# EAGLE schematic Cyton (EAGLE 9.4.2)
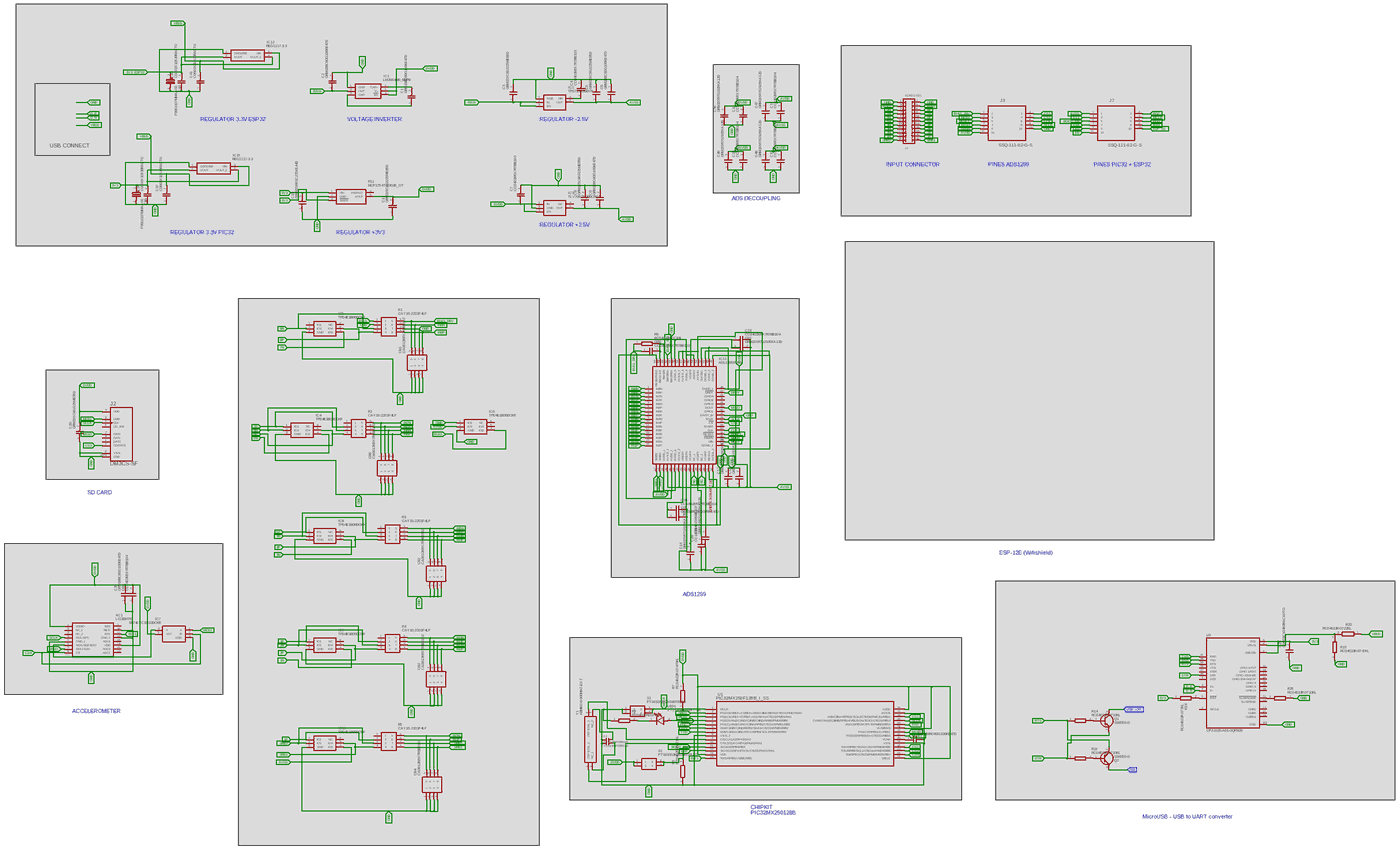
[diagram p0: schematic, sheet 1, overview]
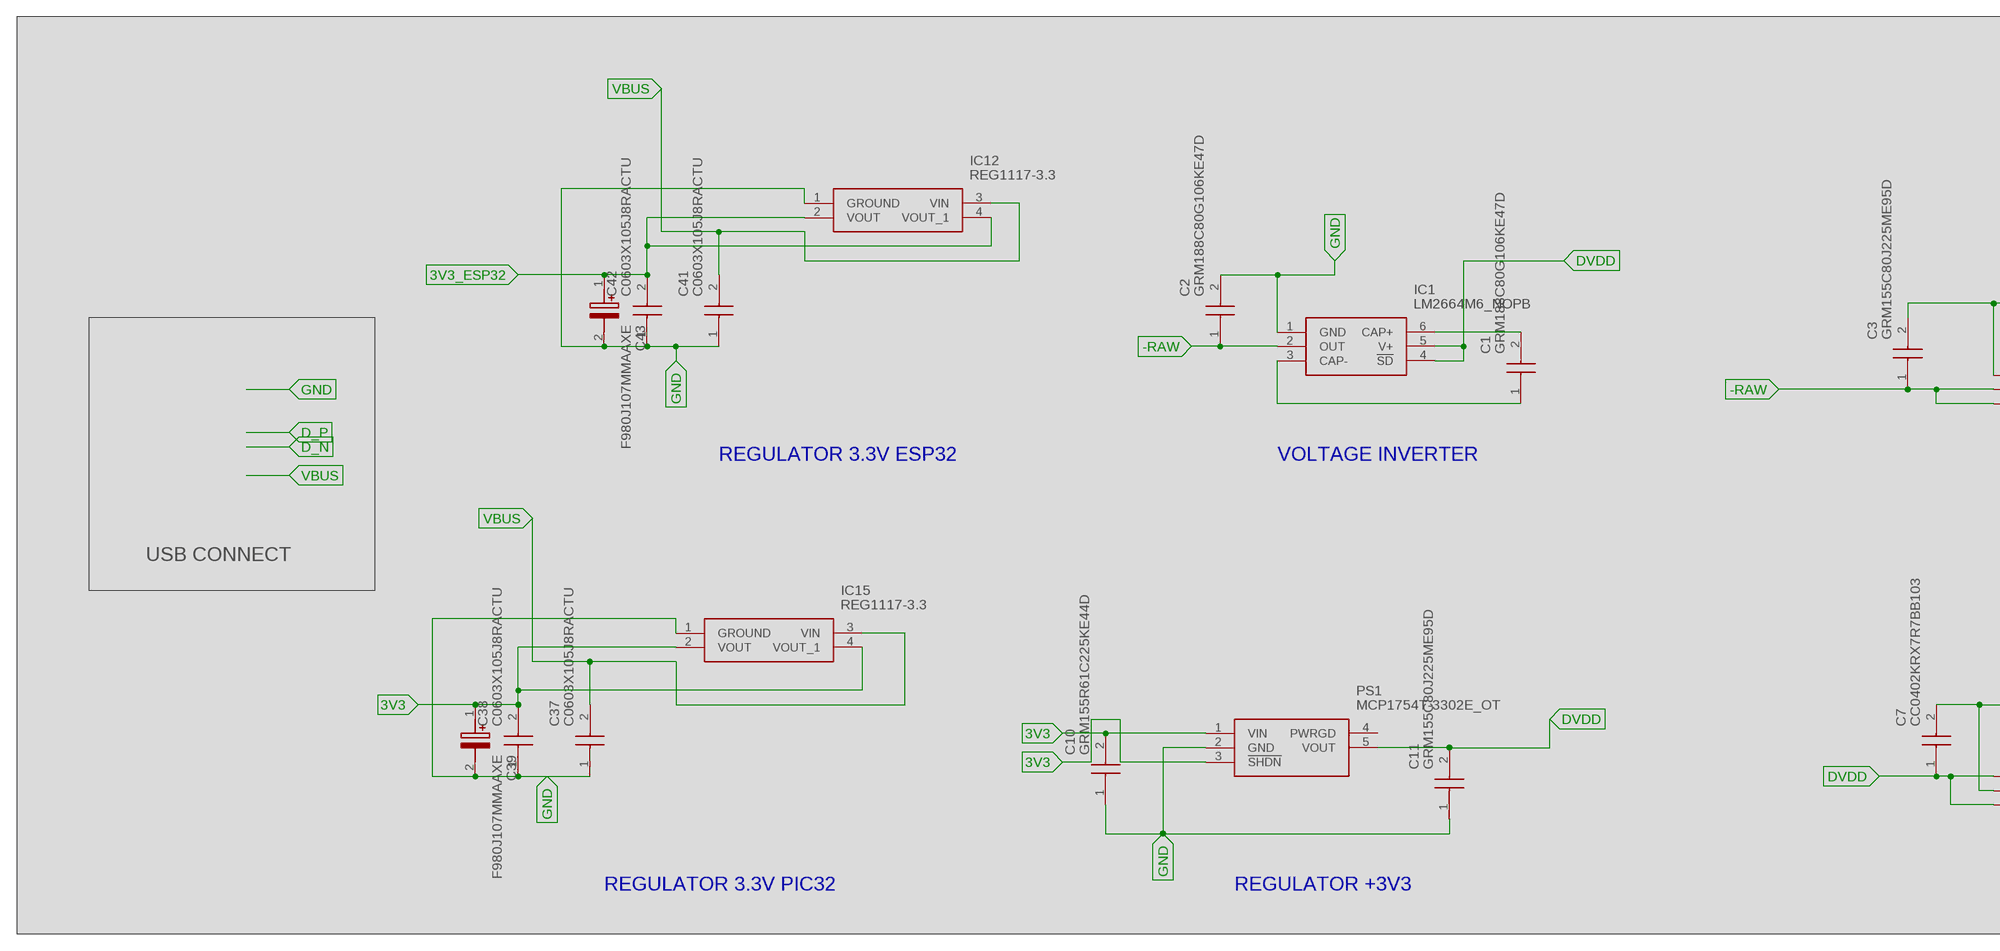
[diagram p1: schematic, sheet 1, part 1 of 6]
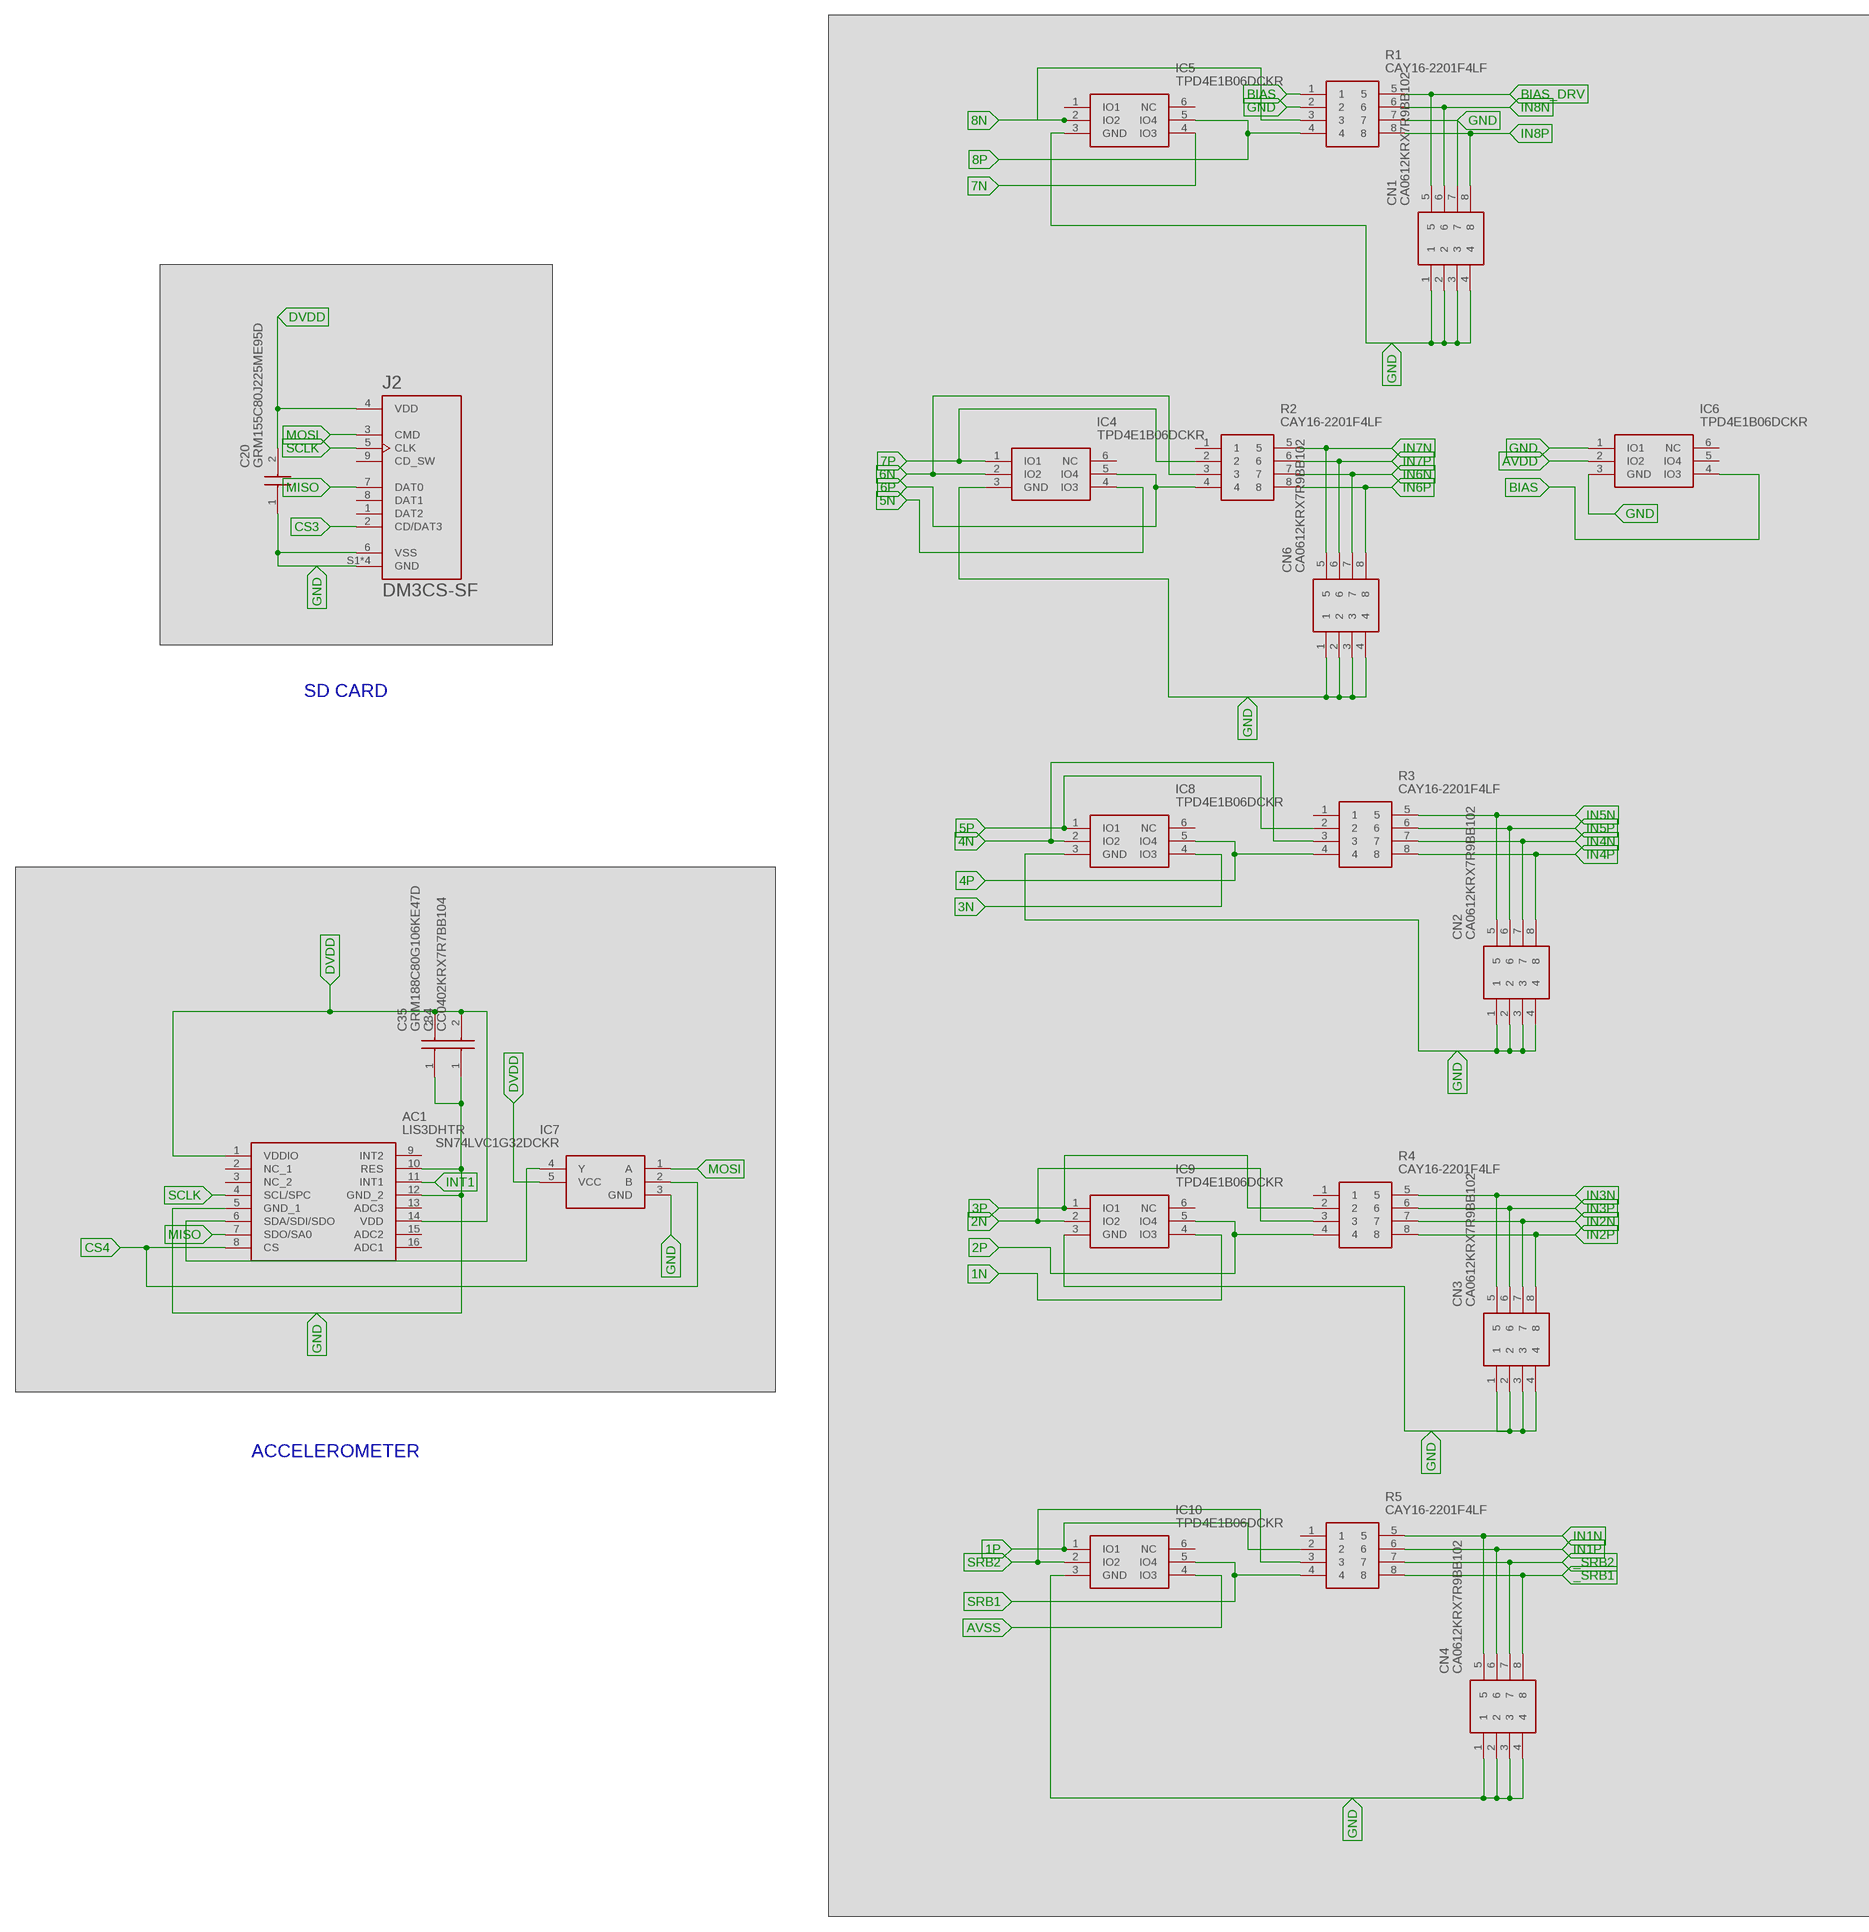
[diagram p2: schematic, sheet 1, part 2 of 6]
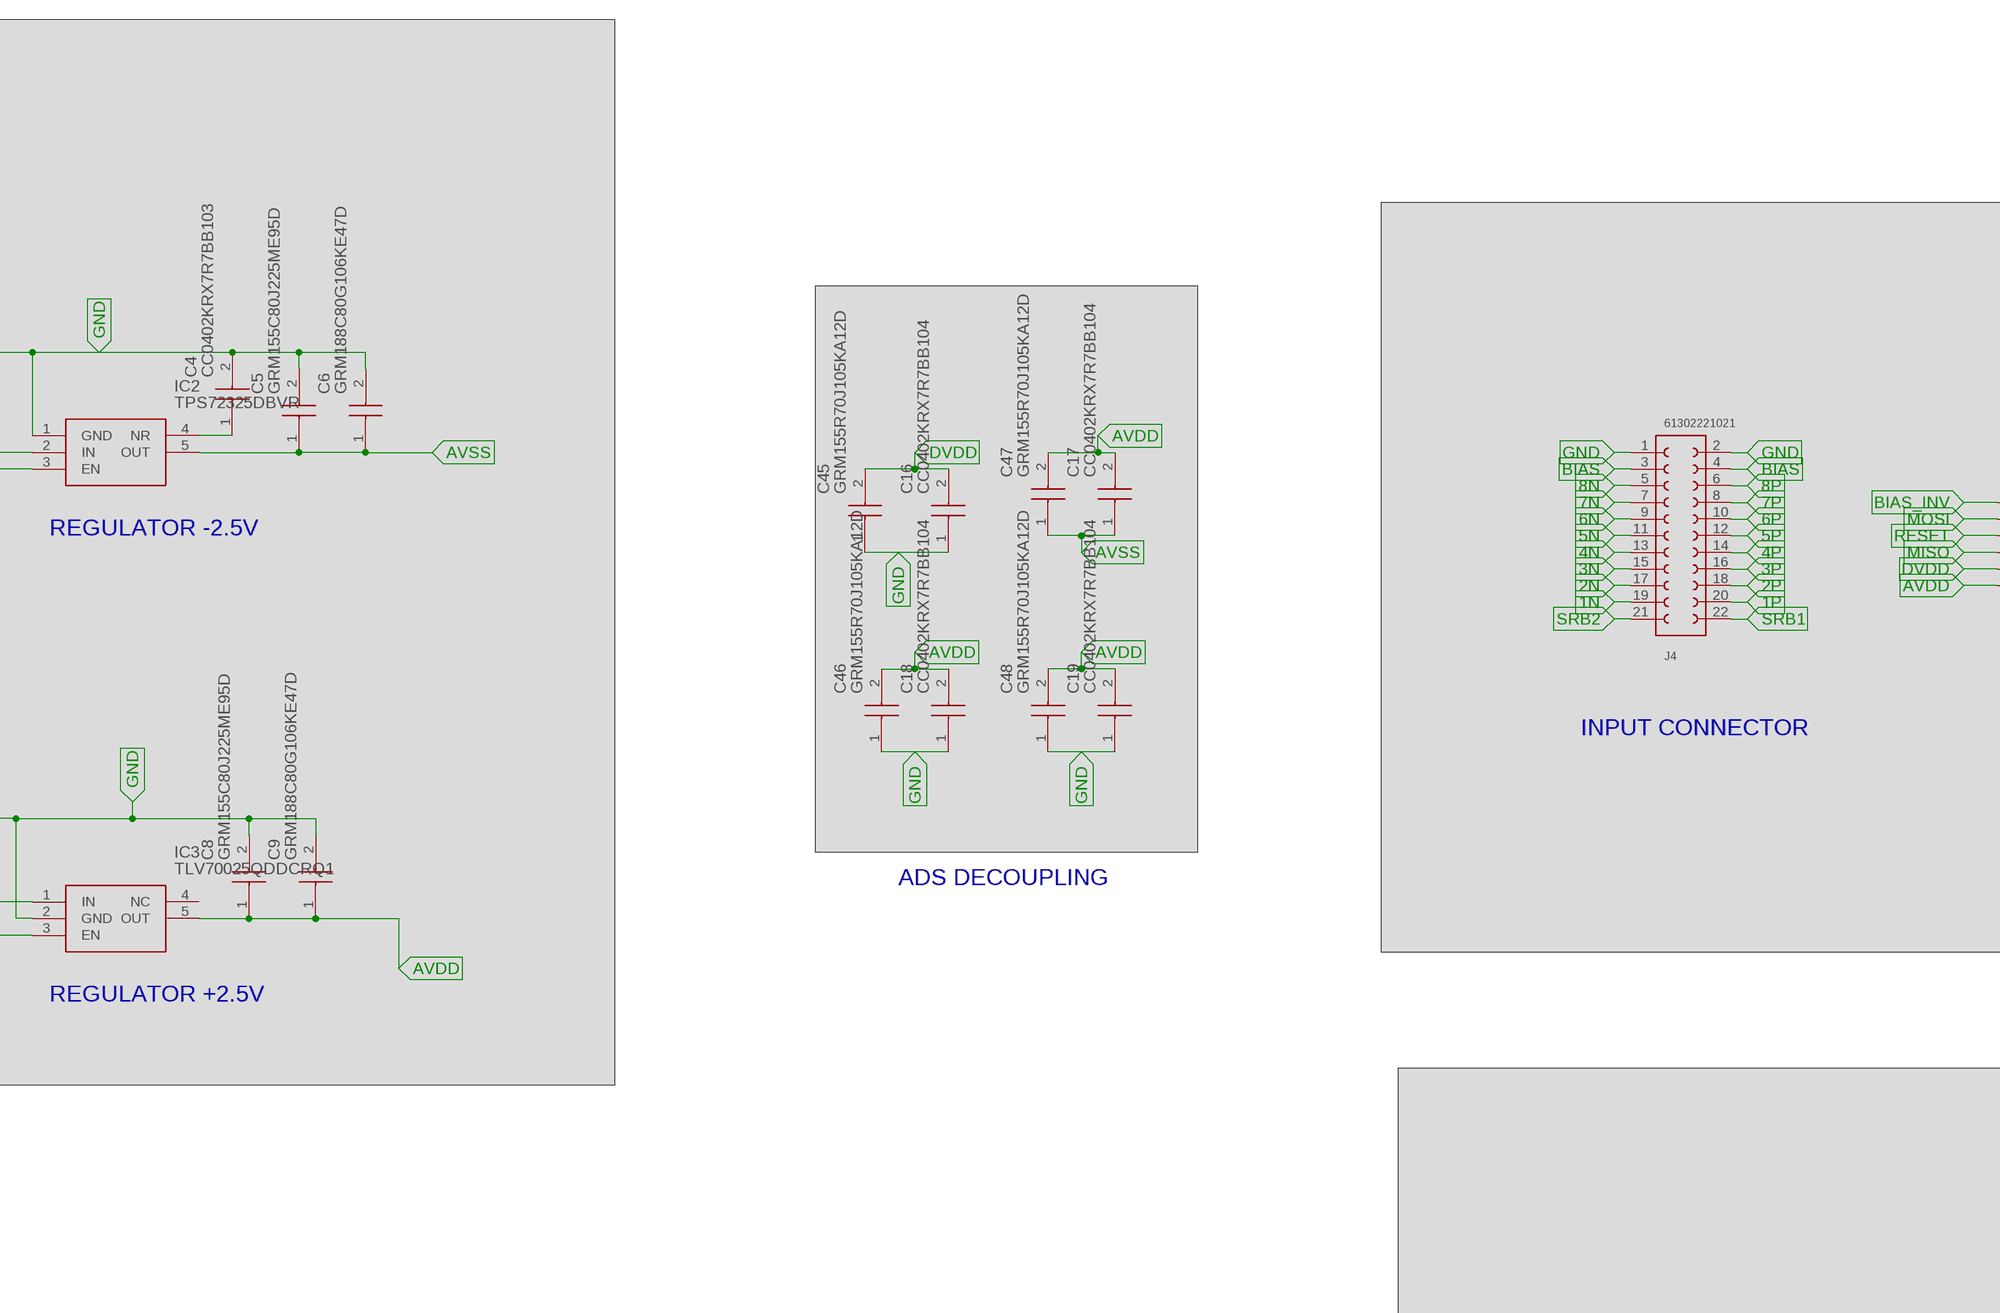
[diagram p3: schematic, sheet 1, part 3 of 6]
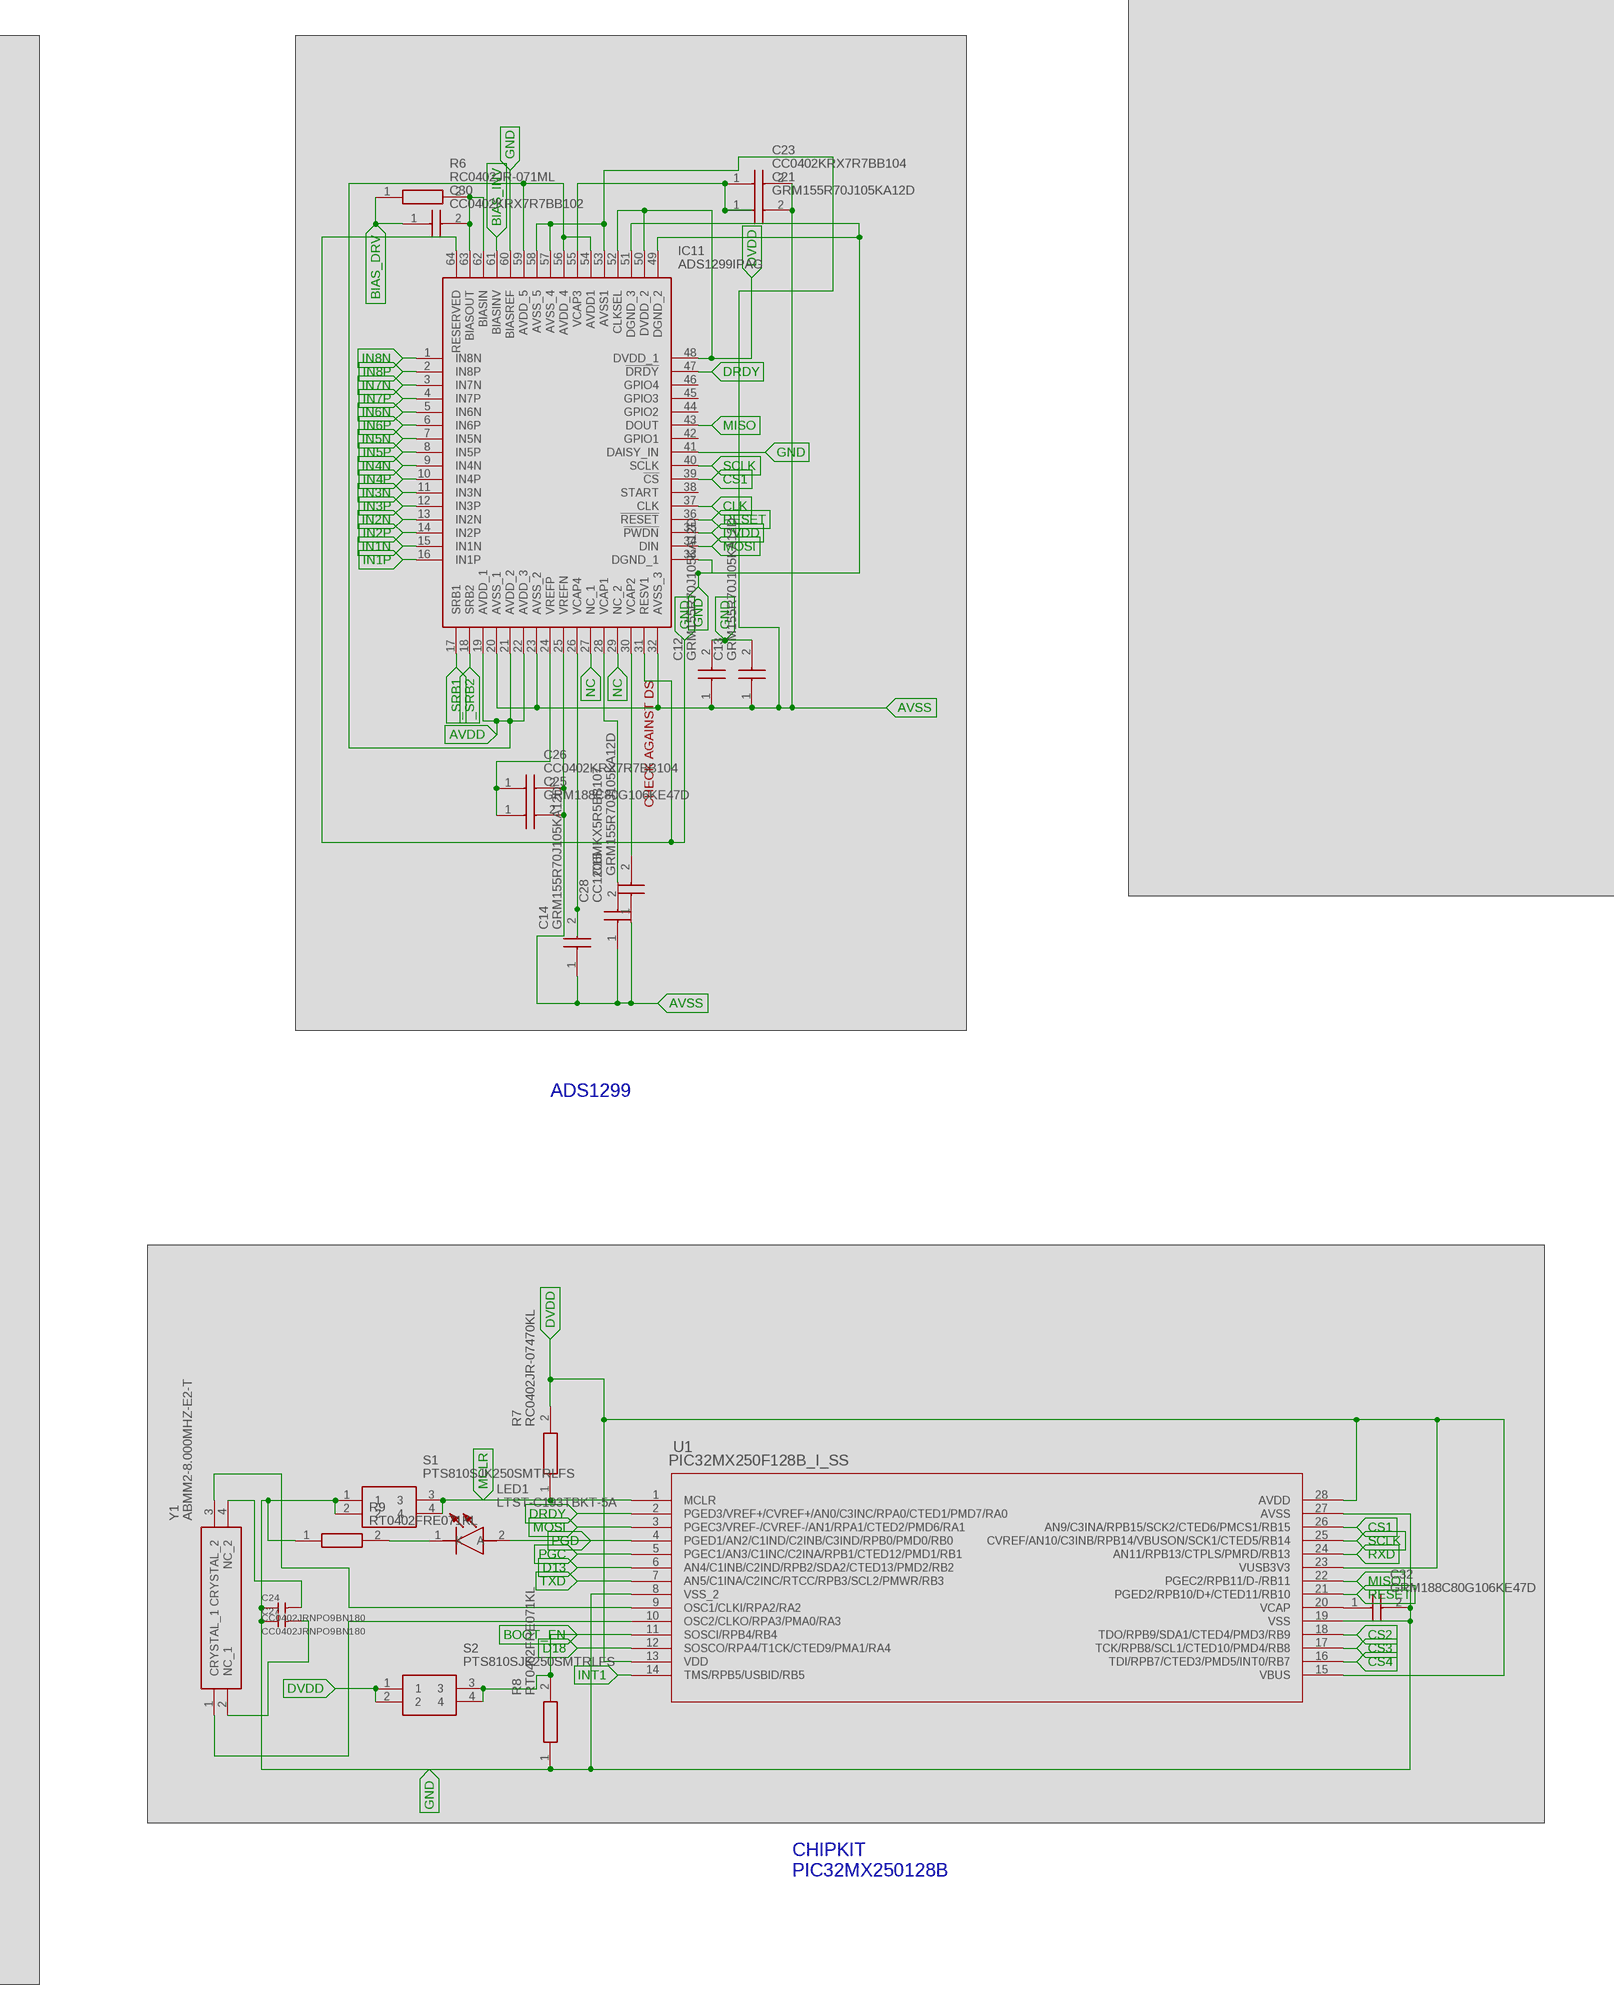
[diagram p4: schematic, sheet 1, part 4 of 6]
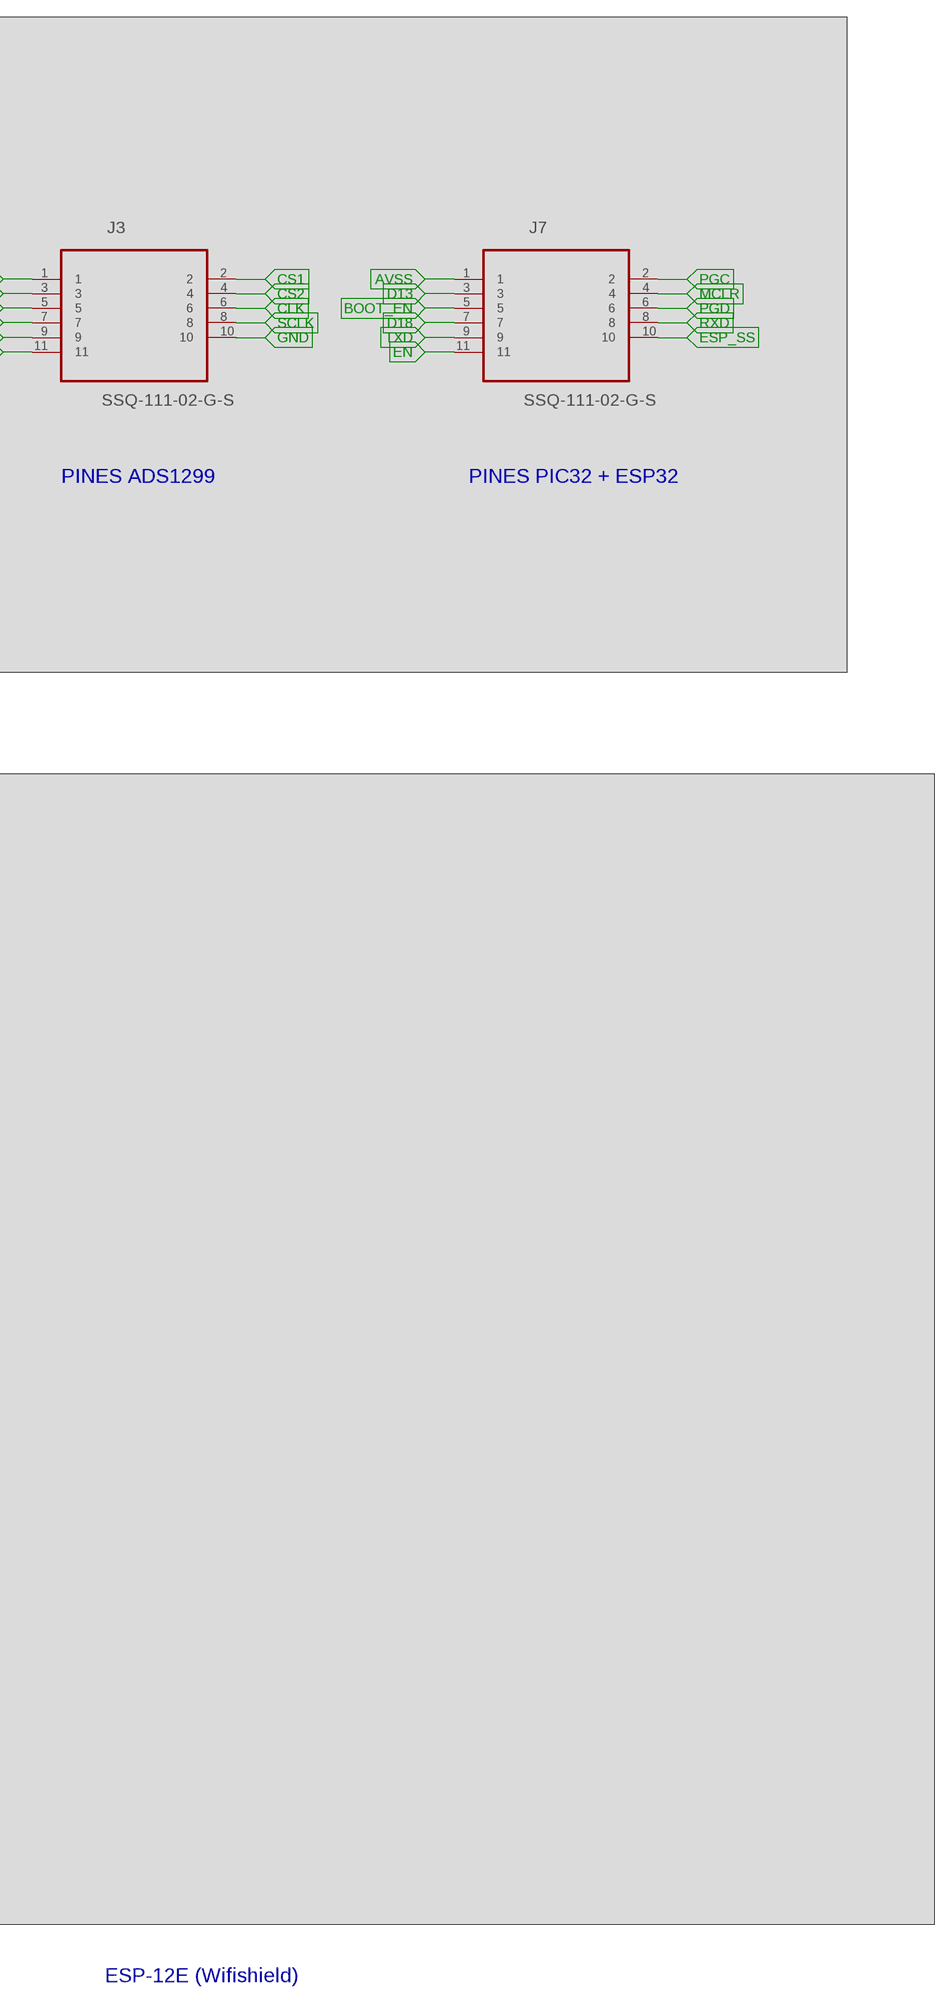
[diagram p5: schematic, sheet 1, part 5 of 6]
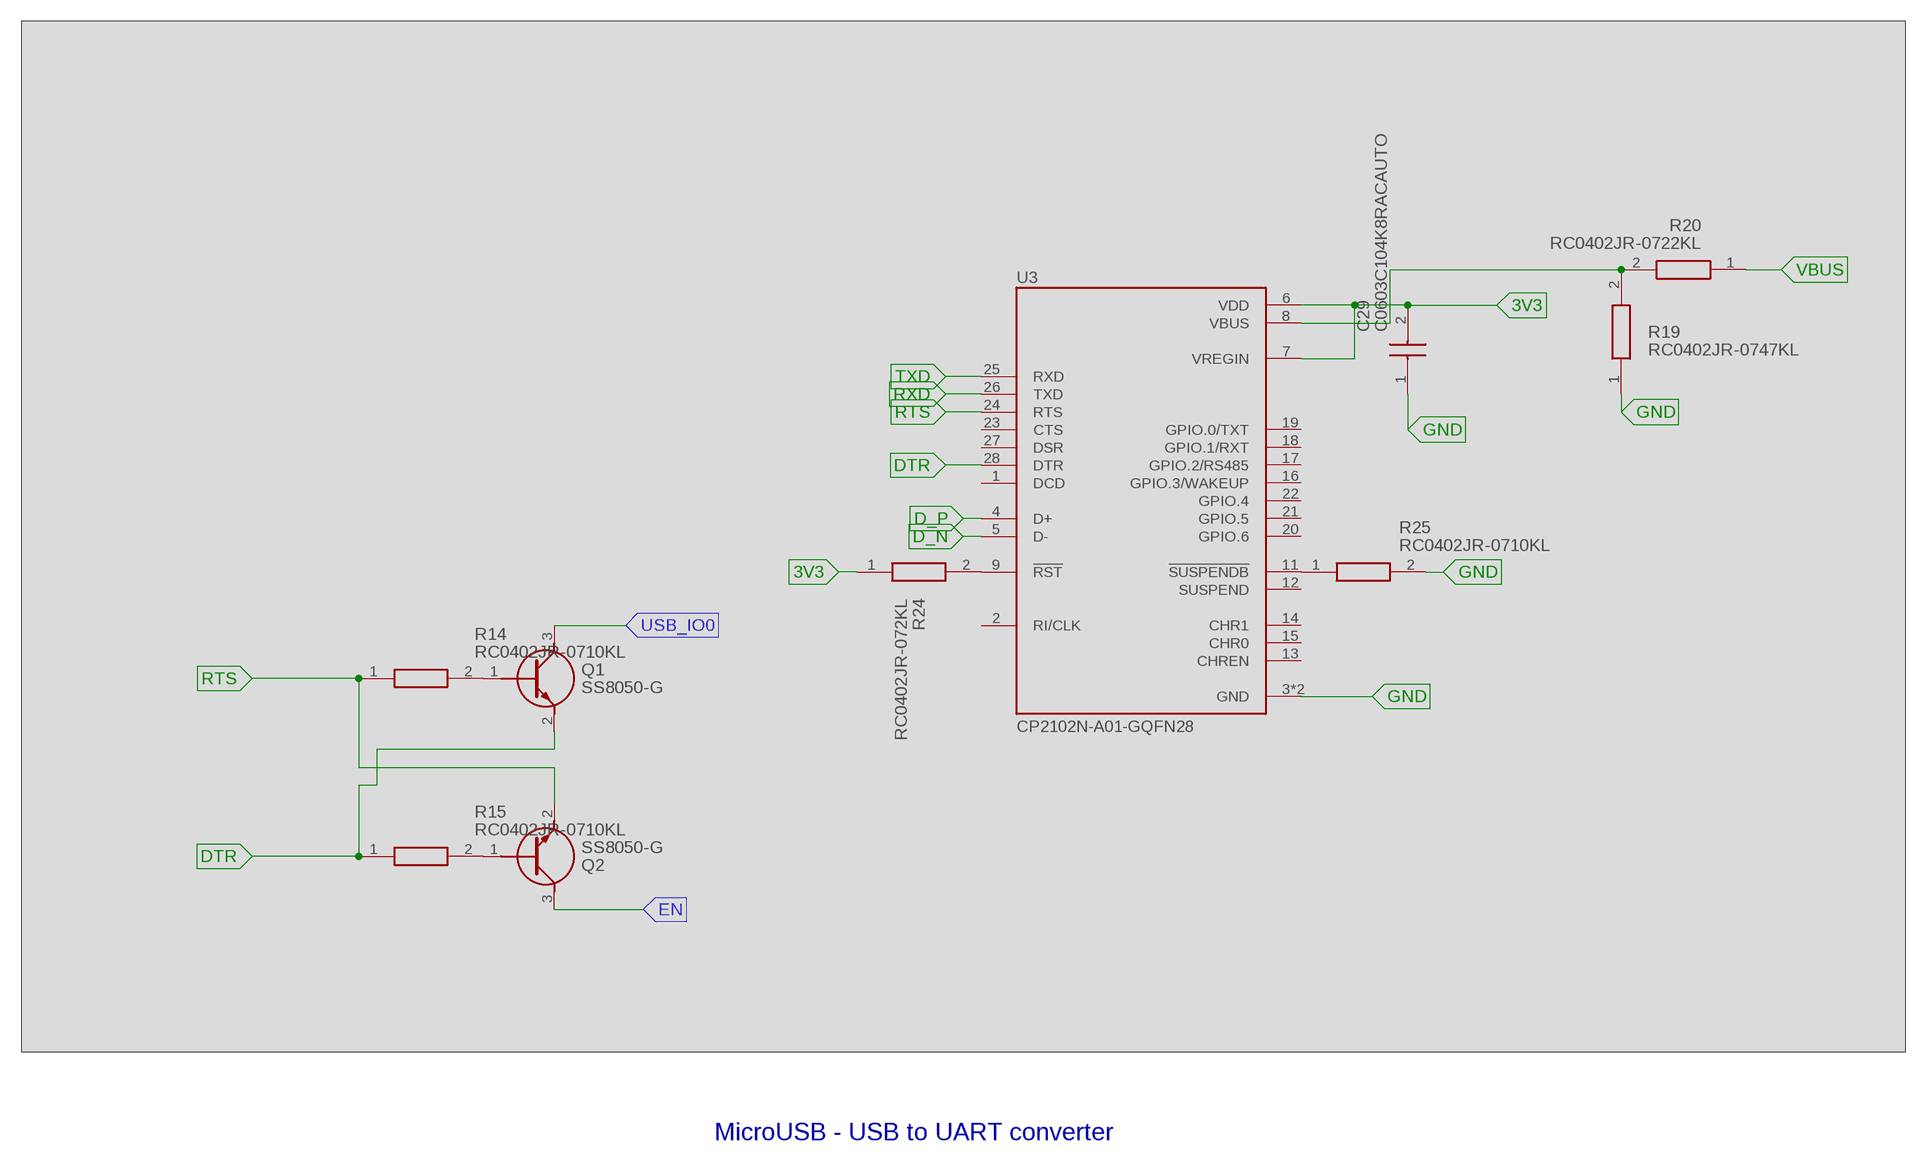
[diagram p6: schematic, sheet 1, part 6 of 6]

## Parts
AC1  LIS3DHTR  [PQFN50P300X300X100-16N]
C1  GRM188C80G106KE47D  [CAPC1608X90N]
C2  GRM188C80G106KE47D  [CAPC1608X90N]
C3  GRM155C80J225ME95D  [CAPC1005X55N]
C4  CC0402KRX7R7BB103  [CAPC1005X55N]
C5  GRM155C80J225ME95D  [CAPC1005X55N]
C6  GRM188C80G106KE47D  [CAPC1608X90N]
C7  CC0402KRX7R7BB103  [CAPC1005X55N]
C8  GRM155C80J225ME95D  [CAPC1005X55N]
C9  GRM188C80G106KE47D  [CAPC1608X90N]
C10  GRM155R61C225KE44D  [CAPC1005X55N]
C11  GRM155C80J225ME95D  [CAPC1005X55N]
C12  GRM155R70J105KA12D  [CAPC1005X55N]
C13  GRM155R70J105KA12D  [CAPC1005X55N]
C14  GRM155R70J105KA12D  [CAPC1005X55N]
C15  GRM155R70J105KA12D  [CAPC1005X55N]
C16  CC0402KRX7R7BB104  [CAPC1005X55N]
C17  CC0402KRX7R7BB104  [CAPC1005X55N]
C18  CC0402KRX7R7BB104  [CAPC1005X55N]
C19  CC0402KRX7R7BB104  [CAPC1005X55N]
C20  GRM155C80J225ME95D  [CAPC1005X55N]
C21  GRM155R70J105KA12D  [CAPC1005X55N]
C23  CC0402KRX7R7BB104  [CAPC1005X55N]
C24  CC0402JRNPO9BN180  [C0402]
C25  GRM188C80G106KE47D  [CAPC1608X90N]
C26  CC0402KRX7R7BB104  [CAPC1005X55N]
C27  CC0402JRNPO9BN180  [C0402]
C28  CC1206MKX5R5BB107  [CAPC3216X125N]
C29  C0603C104K8RACAUTO  [CAPC1608X95N]
C30  CC0402KRX7R7BB102  [CAPC1005X55N]
C32  GRM188C80G106KE47D  [CAPC1608X90N]
C34  CC0402KRX7R7BB104  [CAPC1005X55N]
C35  GRM188C80G106KE47D  [CAPC1608X90N]
C37  C0603X105J8RACTU  [CAPC1608X95N]
C38  C0603X105J8RACTU  [CAPC1608X95N]
C39  F980J107MMAAXE  [CAPPM169X100N]
C41  C0603X105J8RACTU  [CAPC1608X95N]
C42  C0603X105J8RACTU  [CAPC1608X95N]
C43  F980J107MMAAXE  [CAPPM169X100N]
C45  GRM155R70J105KA12D  [CAPC1005X55N]
C46  GRM155R70J105KA12D  [CAPC1005X55N]
C47  GRM155R70J105KA12D  [CAPC1005X55N]
C48  GRM155R70J105KA12D  [CAPC1005X55N]
CN1  CA0612KRX7R9BB102  [CA0612KRX7R9BB102]
CN2  CA0612KRX7R9BB102  [CA0612KRX7R9BB102]
CN3  CA0612KRX7R9BB102  [CA0612KRX7R9BB102]
CN4  CA0612KRX7R9BB102  [CA0612KRX7R9BB102]
CN6  CA0612KRX7R9BB102  [CA0612KRX7R9BB102]
IC1  LM2664M6_NOPB  [SOT95P280X145-6N]
IC2  TPS72325DBVR  [SOT95P280X145-5N]
IC3  TLV70025QDDCRQ1  [SOT95P280X110-5N]
IC4  TPD4E1B06DCKR  [SOT65P210X110-6N]
IC5  TPD4E1B06DCKR  [SOT65P210X110-6N]
IC6  TPD4E1B06DCKR  [SOT65P210X110-6N]
IC7  SN74LVC1G32DCKR  [SOT65P210X110-5N]
IC8  TPD4E1B06DCKR  [SOT65P210X110-6N]
IC9  TPD4E1B06DCKR  [SOT65P210X110-6N]
IC10  TPD4E1B06DCKR  [SOT65P210X110-6N]
IC11  ADS1299IPAG  [QFP50P1200X1200X120-64N]
IC12  REG1117-3.3  [SOT230P700X180-4N]
IC15  REG1117-3.3  [SOT230P700X180-4N]
J2  DM3CS-SF  [HRS_DM3CS-SF]
J3  SSQ-111-02-G-S  [SAMTEC_SSQ-111-02-G-S]
J4  61302221021  [61302221021]
J7  SSQ-111-02-G-S  [SAMTEC_SSQ-111-02-G-S]
LED1  LTST-C193TBKT-5A  [LEDC1608X45N]
PS1  MCP1754T-3302E_OT  [SOT95P270X145-5N]
Q1  SS8050-G  [SOT95P240X115-3N]
Q2  SS8050-G  [SOT95P240X115-3N]
R1  CAY16-2201F4LF  [RESCAX80P160X320X60-8N]
R2  CAY16-2201F4LF  [RESCAX80P160X320X60-8N]
R3  CAY16-2201F4LF  [RESCAX80P160X320X60-8N]
R4  CAY16-2201F4LF  [RESCAX80P160X320X60-8N]
R5  CAY16-2201F4LF  [RESCAX80P160X320X60-8N]
R6  RC0402JR-071ML  [RESC1005X40N]
R7  RC0402JR-07470KL  [RESC1005X40N]
R8  RT0402FRE071KL  [RESC1005X35N]
R9  RT0402FRE071KL  [RESC1005X35N]
R14  RC0402JR-0710KL  [RESC1005X40N]
R15  RC0402JR-0710KL  [RESC1005X40N]
R19  RC0402JR-0747KL  [RESC1005X40N]
R20  RC0402JR-0722KL  [RESC1005X40N]
R24  RC0402JR-072KL  [RESC1005X40N]
R25  RC0402JR-0710KL  [RESC1005X40N]
S1  PTS810SJK250SMTRLFS  [PTS810SJG250SMTRLFS]
S2  PTS810SJK250SMTRLFS  [PTS810SJG250SMTRLFS]
U1  PIC32MX250F128B_I_SS  [SSOP28_MC]
U3  CP2102N-A01-GQFN28  [QFN50P500X500X80-29N]
Y1  ABMM2-8.000MHZ-E2-T  [ABMM2]

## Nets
1N: IC9.4(IO3) J4.19
1P: IC10.1(IO1) J4.20 R5.2
2N: IC9.2(IO2) J4.17 R4.3
2P: IC9.5(IO4) J4.18 R4.4
3N: IC8.4(IO3) J4.15
3P: IC9.1(IO1) J4.16 R4.2
3V3: C10.2 C29.2 C38.2 C39.1(+) IC15.2(VOUT) IC15.4(VOUT_1) PS1.1(VIN) PS1.3(!SHDN) R24.1 U3.6(VDD) U3.7(VREGIN)
3V3_ESP32: C42.2 C43.1(+) IC12.2(VOUT) IC12.4(VOUT_1)
4N: IC8.2(IO2) J4.13 R3.3
4P: IC8.5(IO4) J4.14 R3.4
5N: IC4.4(IO3) J4.11
5P: IC8.1(IO1) J4.12 R3.2
6N: IC4.2(IO2) J4.9 R2.3
6P: IC4.5(IO4) J4.10 R2.4
7N: IC5.4(IO3) J4.7
7P: IC4.1(IO1) J4.8 R2.2
8N: IC5.2(IO2) J4.5 R1.3
8P: IC5.5(IO4) J4.6 R1.4
-RAW: C2.1 C3.1 IC1.2(OUT) IC2.2(IN) IC2.3(EN)
_SRB1: CN4.8 IC11.17(SRB1) R5.8
_SRB2: CN4.7 IC11.18(SRB2) R5.7
AVDD: C8.1 C9.1 C17.2 C18.2 C19.2 C46.2 C47.2 C48.2 IC3.5(OUT) IC6.2(IO2) IC11.19(AVDD_1) IC11.21(AVDD_2) IC11.22(AVDD_3) IC11.54(AVDD1) IC11.56(AVDD_4) IC11.59(AVDD_5) J3.11
AVSS: C5.1 C6.1 C12.1 C13.1 C14.1 C15.1 C17.1 C21.2 C23.2 C25.2 C26.2 C28.1 C47.1 IC2.5(OUT) IC10.4(IO3) IC11.20(AVSS_1) IC11.23(AVSS_2) IC11.25(VREFN) IC11.32(AVSS_3) IC11.53(AVSS1) IC11.57(AVSS_4) IC11.58(AVSS_5) J7.1
BIAS: IC6.4(IO3) J4.3 J4.4 R1.1
BIAS_DRV: C30.1 CN1.5 R1.5 R6.1
BIAS_INV: IC11.61(BIASINV) J3.1
BOOT_EN: J7.5 R8.2 S2.3 S2.4 U1.11(SOSCI/RPB4/RB4)
CLK: IC11.37(CLK) J3.6
CS1: IC11.39(!CS) J3.2 U1.26(AN9/C3INA/RPB15/SCK2/CTED6/PMCS1/RB15)
CS2: J3.4 U1.18(TDO/RPB9/SDA1/CTED4/PMD3/RB9)
CS3: J2.2(CD/DAT3) U1.17(TCK/RPB8/SCL1/CTED10/PMD4/RB8)
CS4: AC1.8(CS) IC7.2(B) U1.16(TDI/RPB7/CTED3/PMD5/INT0/RB7)
D13: J7.3 U1.6(AN4/C1INB/C2IND/RPB2/SDA2/CTED13/PMD2/RB2)
D18: J7.7 U1.12(SOSCO/RPA4/T1CK/CTED9/PMA1/RA4)
D_N: U3.5(D-)
D_P: U3.4(D+)
DRDY: IC11.47(!DRDY) U1.2(PGED3/VREF+/CVREF+/AN0/C3INC/RPA0/CTED1/PMD7/RA0)
DTR: Q1.2(E) R15.1 U3.28(DTR)
DVDD: AC1.1(VDDIO) AC1.14(VDD) C7.1(C1) C11.2 C16.2 C20.2 C34.2 C35.2 C45.2 IC1.4(!SD) IC1.5(V+) IC3.1(IN) IC3.3(EN) IC7.5(VCC) IC11.35(!PWDN) IC11.48(DVDD_1) IC11.50(DVDD_2) IC11.52(CLKSEL) J2.4(VDD) J3.9 PS1.5(VOUT) R7.2 S2.1 S2.2 U1.13(VDD) U1.15(VBUS) U1.23(VUSB3V3) U1.28(AVDD)
EN: J7.11 Q2.3(C)
ESP_SS: J7.10
GND: AC1.5(GND_1) AC1.10(RES) AC1.12(GND_2) C2.2 C3.2 C4.2(C2) C5.2 C6.2 C7.2(C2) C8.2 C9.2 C10.1 C11.1 C12.2 C13.2 C16.1 C18.1 C19.1 C20.1 C24.1 C27.1 C29.1 C32.2 C34.1 C35.1 C37.1 C38.1 C39.2(-) C41.1 C42.1 C43.2(-) C45.1 C46.1 C48.1 CN1.1 CN1.2 CN1.3 CN1.4 CN2.1 CN2.2 CN2.3 CN2.4 CN3.1 CN3.2 CN3.3 CN3.4 CN4.1 CN4.2 CN4.3 CN4.4 CN6.1 CN6.2 CN6.3 CN6.4 IC1.1(GND) IC2.1(GND) IC3.2(GND) IC4.3(GND) IC5.3(GND) IC6.1(IO1) IC6.3(GND) IC7.3(GND) IC8.3(GND) IC9.3(GND) IC10.3(GND) IC11.31(RESV1) IC11.33(DGND_1) IC11.41(DAISY_IN) IC11.49(DGND_2) IC11.51(DGND_3) IC11.60(BIASREF) IC11.64(RESERVED) IC12.1(GROUND) IC15.1(GROUND) J2.6(VSS) J2.S1(GND) J2.S2(GND) J2.S3(GND) J2.S5(GND) J3.10 J4.1 J4.2 PS1.2(GND) R1.2 R8.1 R9.1 R19.1 R25.2 S1.1 S1.2 U1.8(VSS_2) U1.19(VSS) U1.27(AVSS) U3.3(GND) U3.29(GND)
IN1N: CN4.5 IC11.15(IN1N) R5.5
IN1P: CN4.6 IC11.16(IN1P) R5.6
IN2N: CN3.7 IC11.13(IN2N) R4.7
IN2P: CN3.8 IC11.14(IN2P) R4.8
IN3N: CN3.5 IC11.11(IN3N) R4.5
IN3P: CN3.6 IC11.12(IN3P) R4.6
IN4N: CN2.7 IC11.9(IN4N) R3.7
IN4P: CN2.8 IC11.10(IN4P) R3.8
IN5N: CN2.5 IC11.7(IN5N) R3.5
IN5P: CN2.6 IC11.8(IN5P) R3.6
IN6N: CN6.7 IC11.5(IN6N) R2.7
IN6P: CN6.8 IC11.6(IN6P) R2.8
IN7N: CN6.5 IC11.3(IN7N) R2.5
IN7P: CN6.6 IC11.4(IN7P) R2.6
IN8N: CN1.6 IC11.1(IN8N) R1.6
IN8P: CN1.8 IC11.2(IN8P) R1.8
INT1: AC1.11(INT1) U1.14(TMS/RPB5/USBID/RB5)
MCLR: J7.4 R7.1 S1.3 S1.4 U1.1(MCLR)
MISO: AC1.7(SDO/SA0) IC11.43(DOUT) J2.7(DAT0) J3.7 U1.22(PGEC2/RPB11/D-/RB11)
MOSI: IC7.1(A) IC11.34(DIN) J2.3(CMD) J3.3 U1.3(PGEC3/VREF-/CVREF-/AN1/RPA1/CTED2/PMD6/RA1)
N$1: Q2.1(B) R15.2
N$2: C4.1(C1) IC2.4(NR)
N$3: R25.1 U3.11(!SUSPENDB)
N$4: C1.2 IC1.6(CAP+)
N$5: C1.1 IC1.3(CAP-)
N$6: C27.2 Y1.2(NC_1)
N$7: AC1.6(SDA/SDI/SDO) IC7.4(Y)
N$10: Q1.1(B) R14.2
N$11: C24.2 Y1.4(NC_2)
N$12: CN1.7 R1.7
N$15: U1.9(OSC1/CLKI/RPA2/RA2) Y1.3(CRYSTAL_2)
N$16: U1.10(OSC2/CLKO/RPA3/PMA0/RA3) Y1.1(CRYSTAL_1)
N$17: R19.2 R20.2 U3.8(VBUS)
N$18: C32.1 U1.20(VCAP)
N$19: R24.2 U3.9(!RST)
N$32: LED1.1(K) R9.2
N$36: C21.1 C23.1 IC11.55(VCAP3)
N$39: C25.1 C26.1 IC11.24(VREFP)
N$42: C28.2 IC11.28(VCAP1)
N$43: C15.2 IC11.30(VCAP2)
N$57: C30.2 IC11.62(BIASIN) IC11.63(BIASOUT) R6.2
N$97: C14.2 IC11.26(VCAP4)
NC: IC11.27(NC_1) IC11.29(NC_2)
PGC: J7.2 U1.5(PGEC1/AN3/C1INC/C2INA/RPB1/CTED12/PMD1/RB1)
PGD: J7.6 LED1.2(A) U1.4(PGED1/AN2/C1IND/C2INB/C3IND/RPB0/PMD0/RB0)
RESET: IC11.36(!RESET) J3.5 U1.21(PGED2/RPB10/D+/CTED11/RB10)
RTS: Q2.2(E) R14.1 U3.24(RTS)
RXD: J7.8 U1.24(AN11/RPB13/CTPLS/PMRD/RB13) U3.26(TXD)
SCLK: AC1.4(SCL/SPC) IC11.40(SCLK) J2.5(CLK) J3.8 U1.25(CVREF/AN10/C3INB/RPB14/VBUSON/SCK1/CTED5/RB14)
SRB1: IC10.5(IO4) J4.22 R5.4
SRB2: IC10.2(IO2) J4.21 R5.3
TXD: J7.9 U1.7(AN5/C1INA/C2INC/RTCC/RPB3/SCL2/PMWR/RB3) U3.25(RXD)
USB_IO0: Q1.3(C)
VBUS: C37.2 C41.2 IC12.3(VIN) IC15.3(VIN) R20.1
Unconnected: AC1.2(NC_1) AC1.3(NC_2) AC1.9(INT2) AC1.13(ADC3) AC1.15(ADC2) AC1.16(ADC1) IC3.4(NC) IC4.6(NC) IC5.1(IO1) IC5.6(NC) IC6.5(IO4) IC6.6(NC) IC8.6(NC) IC9.6(NC) IC10.6(NC) IC11.38(START) IC11.42(GPIO1) IC11.44(GPIO2) IC11.45(GPIO3) IC11.46(GPIO4) J2.1(DAT2) J2.8(DAT1) J2.9(CD_SW) PS1.4(PWRGD) R2.1 R3.1 R4.1 R5.1 U3.1(DCD) U3.2(RI/CLK) U3.12(SUSPEND) U3.13(CHREN) U3.14(CHR1) U3.15(CHR0) U3.16(GPIO.3/WAKEUP) U3.17(GPIO.2/RS485) U3.18(GPIO.1/RXT) U3.19(GPIO.0/TXT) U3.20(GPIO.6) U3.21(GPIO.5) U3.22(GPIO.4) U3.23(CTS) U3.27(DSR)

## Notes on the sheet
- REGULATOR 3.3V ESP32 | VOLTAGE INVERTER | REGULATOR -2.5V
- USB CONNECT
- INPUT CONNECTOR | PINES ADS1299 | PINES PIC32 + ESP32
- ADS DECOUPLING
- REGULATOR +2.5V
- REGULATOR 3.3V PIC32 | REGULATOR +3V3
- CHECK AGAINST DS
- SD CARD
- ESP-12E (Wifishield)
- ADS1299
- ACCELEROMETER
- CHIPKIT
  PIC32MX250128B
- MicroUSB - USB to UART converter

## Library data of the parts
AC1 = Cyton:LIS3DHTR: Accelerometer 3-Axis 2g/16g 1.8V LGA16 STMicroelectronics LIS3DHTR Accelerometer IC, 3-axis, I2C, SPI 1.71 3.6 V, 16-Pin LGA Source: Datasheet; ALLIED_NUMBER: 70521157; DESCRIPTION: Accelerometer 3-Axis 2g/16g 1.8V LGA16 STMicroelectronics LIS3DHTR Accelerometer IC, 3-axis, I2C, SPI 1.71 3.6 V, 16-Pin LGA; HEIGHT: 1mm; MANUFACTURER_NAME: STMicroelectronics; MANUFACTURER_PART_NUMBER: LIS3DHTR; RS_PART_NUMBER: 7931364P; RS_PRICE-STOCK: http://uk.rs-online.com/web/p/products/7931364P
C1 C2 C6 C9 C25 C32 C35 = Cyton:GRM188C80G106KE47D: Multilayer Ceramic Capacitors MLCC - SMD/SMT 0603 10uF 4volts *Derate Voltage/Temp; DESCRIPTION: Multilayer Ceramic Capacitors MLCC - SMD/SMT 0603 10uF 4volts *Derate Voltage/Temp; HEIGHT: 0.9mm; MANUFACTURER_NAME: Murata Electronics; MANUFACTURER_PART_NUMBER: GRM188C80G106KE47D; RS_PART_NUMBER: 1726485; RS_PRICE-STOCK: http://uk.rs-online.com/web/p/products/1726485
C3 C5 C8 C11 C20 = Cyton:GRM155C80J225ME95D: Multilayer Ceramic Capacitors MLCC - SMD/SMT 0402 2.2uF 6.3volts *Derate Voltage/Temp; DESCRIPTION: Multilayer Ceramic Capacitors MLCC - SMD/SMT 0402 2.2uF 6.3volts *Derate Voltage/Temp; HEIGHT: 0.55mm; MANUFACTURER_NAME: Murata Electronics; MANUFACTURER_PART_NUMBER: GRM155C80J225ME95D
C4 C7 = Cyton:CC0402KRX7R7BB103: CAPACITOR, 0402 10nF +/-10% 16V; DESCRIPTION: CAPACITOR, 0402 10nF +/-10% 16V; HEIGHT: mm; MANUFACTURER_NAME: YAGEO (PHYCOMP); MANUFACTURER_PART_NUMBER: CC0402KRX7R7BB103
C10 = Cyton:GRM155R61C225KE44D: Multilayer Ceramic Capacitors MLCC - SMD/SMT 0402 2.2uF 16volts *Derate Voltage/Temp; DESCRIPTION: Multilayer Ceramic Capacitors MLCC - SMD/SMT 0402 2.2uF 16volts *Derate Voltage/Temp; HEIGHT: 0.55mm; MANUFACTURER_NAME: Murata Electronics; MANUFACTURER_PART_NUMBER: GRM155R61C225KE44D
C12-C15 C21 C45-C48 = Cyton:GRM155R70J105KA12D: Multilayer Ceramic Capacitors MLCC - SMD/SMT 0402 1.0uF 6.3volts *Derate Voltage/Temp; DESCRIPTION: Multilayer Ceramic Capacitors MLCC - SMD/SMT 0402 1.0uF 6.3volts *Derate Voltage/Temp; HEIGHT: 0.55mm; MANUFACTURER_NAME: Murata Electronics; MANUFACTURER_PART_NUMBER: GRM155R70J105KA12D; RS_PART_NUMBER: 1138711P; RS_PRICE-STOCK: http://uk.rs-online.com/web/p/products/1138711P
C16-C19 C23 C26 C34 = Cyton:CC0402KRX7R7BB104: Cap 100nF 16V 0402 SMD 10% X7R Phycomp 100nF Multilayer Ceramic Capacitor (MLCC) 16 V dc +/-10% X7R dielectric Standard max op. temp. +125C; DESCRIPTION: Cap 100nF 16V 0402 SMD 10% X7R Phycomp 100nF Multilayer Ceramic Capacitor (MLCC) 16 V dc +/-10% X7R dielectric Standard max op. temp. +125C; HEIGHT: 0.55mm; MANUFACTURER_NAME: YAGEO (PHYCOMP); MANUFACTURER_PART_NUMBER: CC0402KRX7R7BB104; RS_PART_NUMBER: 6169701; RS_PRICE-STOCK: https://uk.rs-online.com/web/p/products/6169701
C24 C27 = Cyton:CC0402JRNPO9BN180: CERAMIC-18PF-50V-5%-NPO(0402); PACKAGE: CC0402JRNPO9BN180
C28 = Cyton:CC1206MKX5R5BB107: Multilayer Ceramic Capacitors MLCC - SMD/SMT FACTORY NOT ACCEPTING ORDERS; DESCRIPTION: Multilayer Ceramic Capacitors MLCC - SMD/SMT FACTORY NOT ACCEPTING ORDERS; HEIGHT: 1.25mm; MANUFACTURER_NAME: YAGEO (PHYCOMP); MANUFACTURER_PART_NUMBER: CC1206MKX5R5BB107
C29 = Cyton:C0603C104K8RACAUTO: KEMET - C0603C104M8RACTU - CAP, 0.1F, 10V, 20%, X7R, 0603; DESCRIPTION: KEMET - C0603C104M8RACTU - CAP, 0.1F, 10V, 20%, X7R, 0603; HEIGHT: 0.95mm; MANUFACTURER_NAME: Kemet; MANUFACTURER_PART_NUMBER: C0603C104M8RACTU
C30 = Cyton:CC0402KRX7R7BB102: YAGEO - CC0402KRX7R7BB102 - CERAMIC CAPACITOR 1000PF, 16V, X7R, 10%, 0402, FULL REEL; DESCRIPTION: YAGEO - CC0402KRX7R7BB102 - CERAMIC CAPACITOR 1000PF, 16V, X7R, 10%, 0402, FULL REEL; HEIGHT: 0.55mm; MANUFACTURER_NAME: YAGEO (PHYCOMP); MANUFACTURER_PART_NUMBER: CC0402KRX7R7BB102
C37 C38 C41 C42 = Cyton:C0603X105J8RACTU: KEMET - C0603X105J8RACTU - CAP, 1F, 10V, 5%, X7R, 0603, REEL; DESCRIPTION: KEMET - C0603X105J8RACTU - CAP, 1F, 10V, 5%, X7R, 0603, REEL; HEIGHT: 0.95mm; MANUFACTURER_NAME: Kemet; MANUFACTURER_PART_NUMBER: C0603X105J8RACTU
C39 C43 = Cyton:F980J107MMAAXE: Cap Tant Solid 100uF 6.3V M CASE 20% (1.6 X 0.85 X 1mm) Inward L SMD 1608-09 10 Ohm 125C T/R; DESCRIPTION: Cap Tant Solid 100uF 6.3V M CASE 20% (1.6 X 0.85 X 1mm) Inward L SMD 1608-09 10 Ohm 125C T/R; HEIGHT: 1mm; MANUFACTURER_NAME: AVX; MANUFACTURER_PART_NUMBER: F980J107MMAAXE
CN1-CN4 CN6 = Cyton:CA0612KRX7R9BB102: Capacitor,ceramic,multilayer,SMT,50V,1pF Source: Datasheet; DESCRIPTION: Capacitor,ceramic,multilayer,SMT,50V,1pF; HEIGHT: mm; MANUFACTURER_NAME: YAGEO (PHYCOMP); MANUFACTURER_PART_NUMBER: CA0612KRX7R9BB102; RS_PART_NUMBER: 6169789; RS_PRICE-STOCK: http://uk.rs-online.com/web/p/products/6169789
IC1 = Cyton:LM2664M6_NOPB: 1.8V to 5.5Vin Switched Capacitor Voltage Converter Source: Datasheet; DESCRIPTION: 1.8V to 5.5Vin Switched Capacitor Voltage Converter; HEIGHT: 1.45mm; MANUFACTURER_NAME: Texas Instruments; MANUFACTURER_PART_NUMBER: LM2664M6/NOPB; RS_PART_NUMBER: 5358792P; RS_PRICE-STOCK: http://uk.rs-online.com/web/p/products/5358792P
IC2 = Cyton:TPS72325DBVR: TEXAS INSTRUMENTS - TPS72325DBVR - LDO, FIXED, -2.5V, 0.2A, SOT-23-5 Source: Datasheet; DESCRIPTION: TEXAS INSTRUMENTS - TPS72325DBVR - LDO, FIXED, -2.5V, 0.2A, SOT-23-5; HEIGHT: 1.45mm; MANUFACTURER_NAME: Texas Instruments; MANUFACTURER_PART_NUMBER: TPS72325DBVR
IC3 = Cyton:TLV70025QDDCRQ1: Automotive 200-mA Low-IQ Low-Dropout Regulator for Portable Devices Source: Datasheet; DESCRIPTION: Automotive 200-mA Low-IQ Low-Dropout Regulator for Portable Devices; HEIGHT: 1.1mm; MANUFACTURER_NAME: Texas Instruments; MANUFACTURER_PART_NUMBER: TLV70025QDDCRQ1
IC4-IC6 IC8-IC10 = Cyton:TPD4E1B06DCKR: Texas Instruments TPD4E1B06DCKR Quad Bi-Directional ESD Protection Array, 45W peak, 6-Pin SC-70 Source: Datasheet; DESCRIPTION: Texas Instruments TPD4E1B06DCKR Quad Bi-Directional ESD Protection Array, 45W peak, 6-Pin SC-70; HEIGHT: 1.1mm; MANUFACTURER_NAME: Texas Instruments; MANUFACTURER_PART_NUMBER: TPD4E1B06DCKR; RS_PART_NUMBER: 8255330P; RS_PRICE-STOCK: http://uk.rs-online.com/web/p/products/8255330P
IC7 = Cyton:SN74LVC1G32DCKR: Single 2-Input Positive-OR Gate Source: Datasheet; DESCRIPTION: Single 2-Input Positive-OR Gate; HEIGHT: mm; MANUFACTURER_NAME: Texas Instruments; MANUFACTURER_PART_NUMBER: SN74LVC1G32DCKR; RS_PART_NUMBER: 1684862; RS_PRICE-STOCK: https://uk.rs-online.com/web/p/products/1684862
IC11 = Cyton:ADS1299IPAG: Low-Noise, 8-Channel, 24-Bit Analog-to-Digital Converter for Biopotential Measurements Source: Datasheet; DESCRIPTION: Low-Noise, 8-Channel, 24-Bit Analog-to-Digital Converter for Biopotential Measurements; HEIGHT: 1.2mm; MANUFACTURER_NAME: Texas Instruments; MANUFACTURER_PART_NUMBER: ADS1299IPAG
IC12 IC15 = Cyton:REG1117-3.3: 800mA,3.3V,LDO Voltage Reg.,REG1117-3.3 Texas Instruments REG1117-3.3, LDO Voltage Regulator, 0.8A, 3.3 V +/-1%, 3.8 15 Vin, 4-Pin SOT-223 Source: Datasheet; DESCRIPTION: 800mA,3.3V,LDO Voltage Reg.,REG1117-3.3 Texas Instruments REG1117-3.3, LDO Voltage Regulator, 0.8A, 3.3 V +/-1%, 3.8 15 Vin, 4-Pin SOT-223; HEIGHT: 1.8mm; MANUFACTURER_NAME: Texas Instruments; MANUFACTURER_PART_NUMBER: REG1117-3.3; RS_PART_NUMBER: 6200852P; RS_PRICE-STOCK: http://uk.rs-online.com/web/p/products/6200852P
J2 = Cyton:DM3CS-SF: CONN MICRO SD CARD HINGED TYPE; AVAILABILITY: Unavailable; DESCRIPTION: Conn Micro SD Card HDR 8 POS 1.1mm Solder RA SMD Embossed T/R 0.5A; MF: Hirose; MP: DM3CS-SF; PACKAGE: None; PRICE: None; SPICEPREFIX: X
J3 J7 = Cyton:SSQ-111-02-G-S: CONN SOCKET, 2.54MM, THT VERT, 11POS; AVAILABILITY: Unavailable; DESCRIPTION: SSQ Series .100 Tiger Buy™ Socket Strip, Square Tail; MF: Samtec; MP: SSQ-111-02-G-S; PACKAGE: None; PRICE: None
J4 = Cyton:61302221021: WR-PHD 2.54mm Angled Dual Pin Header, 22 Pins =>Code : Con_BTB_PHD_2.54_2_61302221021 Details see: http://katalog.we-online.de/en/em/613_0xx_210_21 Created 2014-05-29, Karrer Zheng 2014 (C) Würth Elektronik; AVAILABILITY: Unavailable; DESCRIPTION: WR-PHD 2.54mm Angled Dual Pin Header 22p; MF: Wurth Electronics; MP: 61302221021; PACKAGE: None; PRICE: None
LED1 = Cyton:LTST-C193TBKT-5A: Standard LEDs - SMD Blue 470nm 28mcd 20mA; DESCRIPTION: Standard LEDs - SMD Blue 470nm 28mcd 20mA; HEIGHT: 0.45mm; MANUFACTURER_NAME: Lite-On; MANUFACTURER_PART_NUMBER: LTST-C193TBKT-5A; RS_PART_NUMBER: 6921051; RS_PRICE-STOCK: https://uk.rs-online.com/web/p/products/6921051
PS1 = Cyton:MCP1754T-3302E_OT: MICROCHIP - MCP1754T-3302E/OT - LDO, FIXED, 3.3V, 0.15A, -40 TO 125DEG C Source: Datasheet; ALLIED_NUMBER: 70451943; DESCRIPTION: MICROCHIP - MCP1754T-3302E/OT - LDO, FIXED, 3.3V, 0.15A, -40 TO 125DEG C; HEIGHT: 1.45mm; MANUFACTURER_NAME: Microchip; MANUFACTURER_PART_NUMBER: MCP1754T-3302E/OT
Q1 Q2 = Cyton:SS8050-G: Bipolar Transistors - BJT NPN TRANSISTOR 1.5A 40V Source: Datasheet; DESCRIPTION: Bipolar Transistors - BJT NPN TRANSISTOR 1.5A 40V; HEIGHT: 1.15mm; MANUFACTURER_NAME: Comchip Technology; MANUFACTURER_PART_NUMBER: SS8050-G
R1-R5 = Cyton:CAY16-2201F4LF: Bourns CAY16 Series 2.2k +/-1% Isolated SMT Resistor Array, 4 Resistors, 0.25W total 1206 Package Convex Source: Datasheet; DESCRIPTION: Bourns CAY16 Series 2.2k +/-1% Isolated SMT Resistor Array, 4 Resistors, 0.25W total 1206 Package Convex; HEIGHT: 0.6mm; MANUFACTURER_NAME: Bourns; MANUFACTURER_PART_NUMBER: CAY16-2201F4LF; RS_PART_NUMBER: 7408773P; RS_PRICE-STOCK: http://uk.rs-online.com/web/p/products/7408773P
R6 = Cyton:RC0402JR-071ML: YAGEO RC0402 VALUE1; DESCRIPTION: YAGEO RC0402 VALUE1; HEIGHT: 0.4mm; MANUFACTURER_NAME: YAGEO (PHYCOMP); MANUFACTURER_PART_NUMBER: RC0402JR-071ML
R7 = Cyton:RC0402JR-07470KL: RESISTOR, 0402 470k Ohms +/-5% 1/16 W; DESCRIPTION: RESISTOR, 0402 470k Ohms +/-5% 1/16 W; HEIGHT: 0.4mm; MANUFACTURER_NAME: YAGEO (PHYCOMP); MANUFACTURER_PART_NUMBER: RC0402JR-07470KL
R8 R9 = Cyton:RT0402FRE071KL: Thin Film Resistors - SMD 1K ohm 1% 1/16W; DESCRIPTION: Thin Film Resistors - SMD 1K ohm 1% 1/16W; HEIGHT: 0.35mm; MANUFACTURER_NAME: YAGEO (PHYCOMP); MANUFACTURER_PART_NUMBER: RT0402FRE071KL
R14 R15 R25 = Cyton:RC0402JR-0710KL: YAGEO (PHYCOMP) - RC0402JR-0710KL - RES, THICK FILM, 10K, 5%, 0.0625W, 0402; DESCRIPTION: YAGEO (PHYCOMP) - RC0402JR-0710KL - RES, THICK FILM, 10K, 5%, 0.0625W, 0402; HEIGHT: 0.4mm; MANUFACTURER_NAME: YAGEO (PHYCOMP); MANUFACTURER_PART_NUMBER: RC0402JR-0710KL
R19 = Cyton:RC0402JR-0747KL: YAGEO (PHYCOMP) - RC0402JR-0747KL - RES, THICK FILM, 47K, 5%, 0.063W, 0402; DESCRIPTION: YAGEO (PHYCOMP) - RC0402JR-0747KL - RES, THICK FILM, 47K, 5%, 0.063W, 0402; HEIGHT: 0.4mm; MANUFACTURER_NAME: YAGEO (PHYCOMP); MANUFACTURER_PART_NUMBER: RC0402JR-0747KL
R20 = Cyton:RC0402JR-0722KL: YAGEO (PHYCOMP) - RC0402JR-0722KL - RES, THICK FILM, 22K, 5%, 0.063W, 0402; DESCRIPTION: YAGEO (PHYCOMP) - RC0402JR-0722KL - RES, THICK FILM, 22K, 5%, 0.063W, 0402; HEIGHT: 0.4mm; MANUFACTURER_NAME: YAGEO (PHYCOMP); MANUFACTURER_PART_NUMBER: RC0402JR-0722KL
R24 = Cyton:RC0402JR-072KL: RESISTOR, 0402 2K Ohms +/-5% 1/16 W; DESCRIPTION: RESISTOR, 0402 2K Ohms +/-5% 1/16 W; HEIGHT: 0.4mm; MANUFACTURER_NAME: YAGEO (PHYCOMP); MANUFACTURER_PART_NUMBER: RC0402JR-072KL
S1 S2 = Cyton:PTS810SJK250SMTRLFS: IP40 Black Button Tactile Switch, SPST-NO 50 mA 3mm Surface Mount Source: Datasheet; DESCRIPTION: IP40 Black Button Tactile Switch, SPST-NO 50 mA 3mm Surface Mount; HEIGHT: mm; MANUFACTURER_NAME: C & K COMPONENTS; MANUFACTURER_PART_NUMBER: PTS810SJK250SMTRLFS; RS_PART_NUMBER: 1359396P; RS_PRICE-STOCK: http://uk.rs-online.com/web/p/products/1359396P
U1 = Cyton:PIC32MX250F128B_I_SS; AVAILABILITY: Unavailable; DESCRIPTION: PIC32 Series 32 kB RAM 128 KB Flash 19 I/O 32-Bit Microcontroller - SSOP-28; MF: Microchip; MP: PIC32MX250F128B-I/SS; PACKAGE: SSOP-28 Microchip; PRICE: None
U3 = Cyton:CP2102N-A01-GQFN28: Ic Bridge Usb To Uart 28qfn; AVAILABILITY: Unavailable; DESCRIPTION: Usb-Uart Interface Bridge, Qfn-28; MF: Silicon Labs; MP: CP2102N-A01-GQFN28; PACKAGE: QFN-28 Silicon Labs; PRICE: None
Y1 = Cyton:ABMM2-8.000MHZ-E2-T: Abracon 8MHz Crystal Unit +/-20ppm SMD 4-Pin 6 x 3.6 x 1.2mm Source: Datasheet; DESCRIPTION: Abracon 8MHz Crystal Unit +/-20ppm SMD 4-Pin 6 x 3.6 x 1.2mm; HEIGHT: mm; MANUFACTURER_NAME: ABRACON; MANUFACTURER_PART_NUMBER: ABMM2-8.000MHZ-E2-T; RS_PART_NUMBER: 1712700; RS_PRICE-STOCK: https://uk.rs-online.com/web/p/products/1712700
